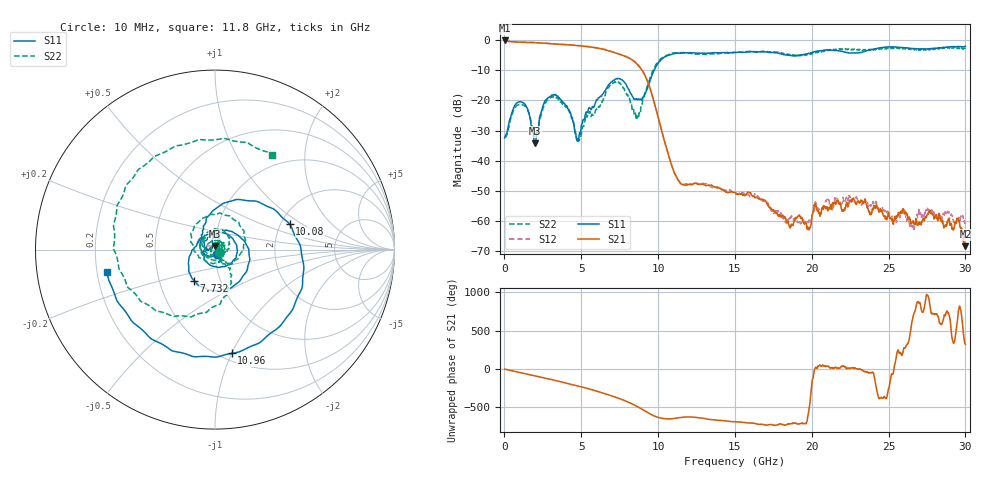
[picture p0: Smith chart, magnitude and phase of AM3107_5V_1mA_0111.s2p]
# Hz S DB R 50.0
!freq dBS11 angS11 dBS21 angS21 dBS12 angS12 dBS22 angS22
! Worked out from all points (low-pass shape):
!   1601 points, 10 MHz to 30 GHz, reference 50 ohm
!   highest |S21| = -0.13 dB at 10 MHz (marker M1); lowest = -68.3 dB at 30 GHz (marker M2)
!   |S21| within 3 dB of the highest: start of sweep to 6.492 GHz
!   lowest |S11| = -34.2 dB at 1.978 GHz (marker M3), VSWR 1.04, Z = 50 + j1.95 ohm
!   |S11| at or under -10 dB: start of sweep to 9.749 GHz
!   |S22| runs from -34.1 to -2.3 dB; largest |S21 - S12| = 0.011
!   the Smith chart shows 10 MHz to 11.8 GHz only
!   S11 on the Smith chart (normalised r, x): 10 MHz: 1.02, -0.04; 7.732 GHz: 0.75, -0.27; 10.08 GHz: 2.24, +0.78; 10.96 GHz: 0.57, -1.00; 11.8 GHz: 0.24, -0.10
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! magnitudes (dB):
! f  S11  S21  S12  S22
! 10 MHz  -32.4  -0.1  -0.1  -32.1
! 1.022 GHz  -20.4  -0.7  -0.6  -21.3
! 1.978 GHz  -34.2  -0.9  -0.8  -32.2
! 2.597 GHz  -20.6  -1.1  -1.0  -21.3
! 3.196 GHz  -18.1  -1.3  -1.2  -18.7
! 4.171 GHz  -23.0  -1.6  -1.5  -23.1
! 4.715 GHz  -33.0  -1.8  -1.7  -33.2
! 5.015 GHz  -28.2  -2.0  -1.9  -30.7
! 6.851 GHz  -14.5  -3.7  -3.6  -15.0
! 7.732 GHz  -13.6  -5.1  -5.0  -16.0
! 8.707 GHz  -19.6  -8.4  -8.2  -26.1
! 10.02 GHz  -7.6  -25.9  -25.8  -7.1
! 10.08 GHz  -7.1  -27.0  -26.9  -6.7
! 10.96 GHz  -4.6  -42.6  -42.6  -4.3
! 11.8 GHz  -4.2  -48.1  -47.8  -4.2
! 15.01 GHz  -4.1  -50.5  -50.9  -4.0
! 18.64 GHz  -5.2  -61.4  -59.1  -4.8
! 20.01 GHz  -4.1  -58.1  -59.1  -4.6
! 22.35 GHz  -4.2  -55.4  -52.9  -3.2
! 25.01 GHz  -2.3  -57.6  -57.4  -2.8
! 29.48 GHz  -2.2  -59.3  -60.5  -2.8
! 30 GHz  -2.1  -68.3  -62.1  -2.5
